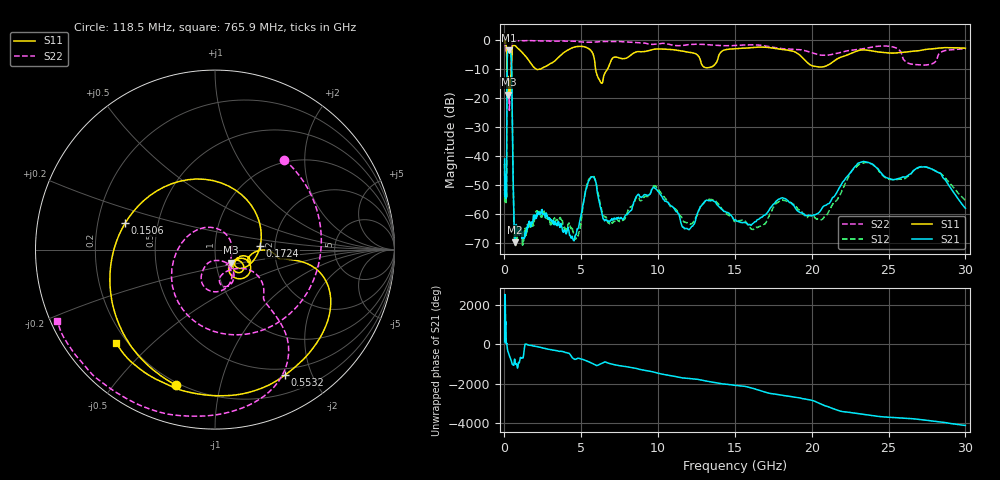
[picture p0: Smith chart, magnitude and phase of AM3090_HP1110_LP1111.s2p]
! Date/Time: Thu, Feb 28, 2019 2:09 PM
! Network Analyzer: Agilent Technologies E8364B Rev: A.07.50.67
! Sweep from 0.010 to 30.000 GHz, 1601 Points, Sweep Type: LOG
! Power Supply: 5.023 V, 0.002 A
# Hz S DB R 50
!freq MagS11 AngS11 MagS21 AngS21 MagS12 AngS12 MagS22 AngS22
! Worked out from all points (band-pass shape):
!   1601 points, 10 MHz to 30 GHz, reference 50 ohm
!   highest |S21| = -3.55 dB at 303.5 MHz (marker M1); lowest = -69.7 dB at 703.4 MHz (marker M2)
!   |S21| within 3 dB of the highest: 179.2 MHz to 444.6 MHz (265.4 MHz wide, 85.1 % of centre)
!   lowest |S11| = -18.9 dB at 262.5 MHz (marker M3), VSWR 1.26, Z = 59 - j8.62 ohm
!   |S11| at or under -10 dB: 165.8 MHz to 436.6 MHz (270.7 MHz wide, 89.9 % of centre); 2.038 GHz to 2.389 GHz (350.8 MHz wide, 15.8 % of centre); 5.929 GHz to 6.719 GHz (789.7 MHz wide, 12.5 % of centre)
!   |S22| runs from -24.3 to -0.2 dB; largest |S21 - S12| = 0.014
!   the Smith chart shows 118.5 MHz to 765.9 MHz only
!   S11 on the Smith chart (normalised r, x): 118.5 MHz: 0.19, -0.74; 150.6 MHz: 0.32, +0.13; 172.4 MHz: 1.67, +0.06; 553.2 MHz: 0.41, -1.62; 765.9 MHz: 0.16, -0.39
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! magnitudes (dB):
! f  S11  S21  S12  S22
! 10 MHz  -0.3  -41.0  -43.1  -0.7
! 18.41 MHz  -1.2  -52.2  -54.8  -1.4
! 38.04 MHz  -0.3  -51.8  -49.1  -1.5
! 118.5 MHz  -2.1  -53.1  -52.7  -4.0
! 144.7 MHz  -4.5  -48.0  -48.7  -5.4
! 150.6 MHz  -5.7  -38.9  -38.5  -6.3
! 172.4 MHz  -12.0  -8.8  -8.7  -20.2
! 262.5 MHz  -18.9  -3.6  -3.6  -15.2
! 303.5 MHz  -14.3  -3.5  -3.5  -21.3
! 450.6 MHz  -8.9  -7.1  -7.1  -8.2
! 550.5 MHz  -2.0  -43.7  -43.5  -0.5
! 553.2 MHz  -1.9  -44.6  -44.3  -0.5
! 703.4 MHz  -2.0  -69.7  -69.3  -0.2
! 765.9 MHz  -2.4  -63.7  -67.1  -0.3
! 2.084 GHz  -10.2  -60.8  -58.9  -0.3
! 4.687 GHz  -2.4  -66.6  -68.2  -0.6
! 5.697 GHz  -4.1  -47.2  -46.9  -0.8
! 7.926 GHz  -6.3  -60.2  -60.5  -0.7
! 9.878 GHz  -3.2  -51.5  -50.5  -1.5
! 20.31 GHz  -9.2  -60.1  -61.7  -4.9
! 23.48 GHz  -3.5  -42.0  -42.3  -2.9
! 30 GHz  -2.9  -58.0  -55.3  -3.1
